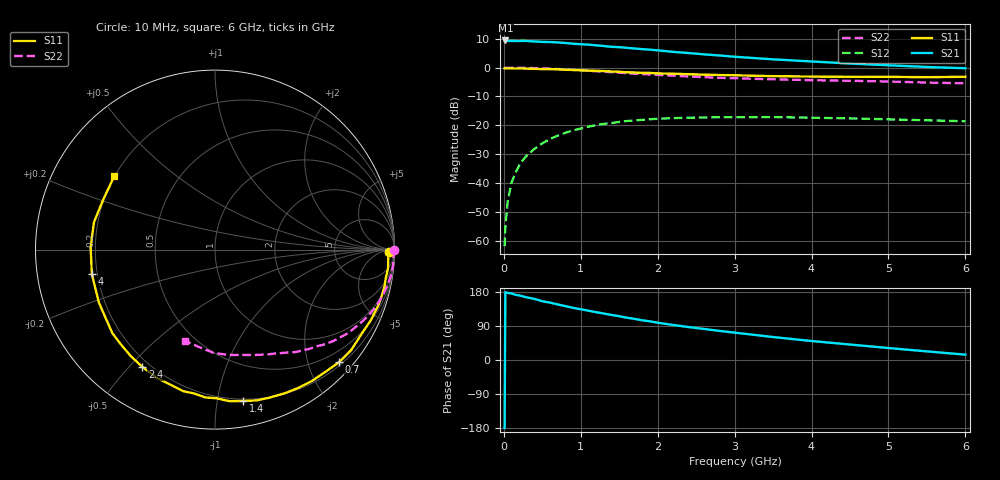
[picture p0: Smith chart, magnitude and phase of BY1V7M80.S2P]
! SIEMENS Small Signal Semiconductors
! BFY420
! Si NPN RF SIEGET Grounded Emitter Transistor in MICRO-X
! VCE = 1.75 V  IC = 0.8 mA
! Common Emitter S-Parameters:  October  1996
# GHz  S  MA  R  50
!  f  S11  S21  S12  S22
! GHz  MAG  ANG  MAG  ANG  MAG  ANG  MAG  ANG
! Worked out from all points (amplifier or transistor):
!   36 points, 10 MHz to 6 GHz, reference 50 ohm
!   highest |S21| = 9.4 dB at 20 MHz (marker M1)
!   |S21| within 3 dB of that: start of sweep to 1.795 GHz
!   unconditionally stable (mu >= 1): 4.667 GHz to end of sweep
!   at 250 MHz: K = 0.03, MSG = 20.6 dB, |S12| = -32.0 dB
!   at 1.4 GHz: K = 0.20, MSG = 13.2 dB, |S12| = -19.2 dB
!   at 6 GHz: K = 1.36, MAG = 5.6 dB, |S12| = -18.6 dB
!   S11 on the Smith chart (normalised r, x): 10 MHz: 51, -26; 700 MHz: 0.26, -2.57; 1.4 GHz: 0.19, -1.19; 2.4 GHz: 0.17, -0.55; 4 GHz: 0.18, -0.09; 6 GHz: 0.20, +0.31
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0.01  0.9695 -0.9  2.956 -179.4  0.0008 101.9  0.9992 -0.2
0.02  0.9677 -1.4  2.96 178.8  0.0017 93.3  0.9924 -0.5
0.05  0.9669 -3.3  2.902 177.0  0.0048 88.5  0.9974 -1.5
0.1  0.9696 -6.3  2.908 175.6  0.0101 87.4  0.9945 -3.0
0.15  0.9647 -9.3  2.899 172.0  0.0149 82.9  0.9959 -4.6
0.2  0.9663 -12.1  2.894 170.4  0.0201 83.0  0.9947 -6.0
0.3  0.9624 -18.2  2.896 165.1  0.03 79.5  0.9886 -9.2
0.4  0.953 -24.4  2.845 161.1  0.0392 75.2  0.9795 -12.1
0.5  0.942 -30.4  2.795 155.1  0.0485 71.0  0.9696 -15.1
0.7  0.9338 -42.2  2.736 146.7  0.066 64.0  0.9445 -20.7
0.9  0.9097 -53.4  2.598 137.6  0.0816 56.6  0.9136 -25.9
1.1  0.8896 -64.2  2.507 130.0  0.0945 50.3  0.8818 -30.9
1.4  0.858 -79.4  2.295 118.9  0.1096 41.4  0.8343 -37.5
1.8  0.8101 -98.2  2.093 104.7  0.1242 31.2  0.7731 -44.9
2.2  0.7847 -114.6  1.877 92.5  0.1331 22.5  0.727 -51.7
2.4  0.7689 -121.7  1.791 86.9  0.1353 19.2  0.7018 -54.8
2.8  0.7441 -135.0  1.625 76.9  0.1379 12.5  0.6665 -60.4
3.5  0.7111 -155.5  1.393 60.6  0.1386 3.8  0.6272 -69.4
4  0.6995 -168.8  1.279 50.1  0.1353 -0.9  0.6049 -76.0
4.5  0.6929 179.0  1.178 40.8  0.1317 -4.9  0.5915 -83.0
5.5  0.6825 155.2  1.027 22.7  0.122 -9.0  0.5509 -99.0
6  0.6936 144.0  0.976 14.1  0.1175 -8.9  0.5339 -108.2
